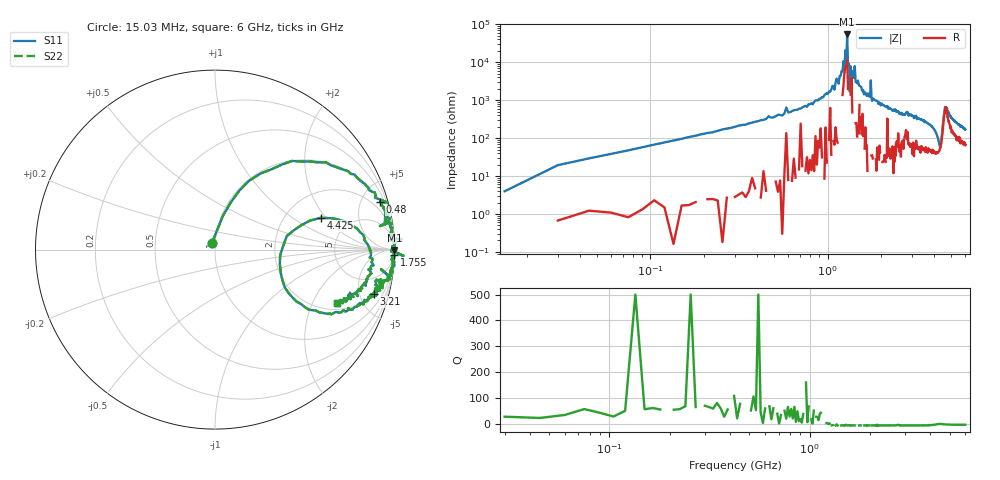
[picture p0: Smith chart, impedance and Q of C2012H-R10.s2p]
!	Network	Analyzer	HP8753E.07.74:	Oct	30	2002	Serial	No.	JP38451487
!	Hewlett-Packard
!	28	Aug	2009	10:31:47
!	Frequency	S11	S21	S12	S22
#	HZ	S	RI	R	50
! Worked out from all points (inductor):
!   400 points, 15.03 MHz to 6 GHz, reference 50 ohm
!   read as one part in series: L = 102 nH near 45.03 MHz
!   highest |Z| = 54.3 kohm at 1.29 GHz (marker M1)
!   self-resonance near 1.26 GHz
!   S11 on the Smith chart (normalised r, x): 15.03 MHz: 0.96, +0.07; 480 MHz: 1.10, +6.94; 1.755 GHz: 1, -67; 3.21 GHz: 2.08, -6.68; 4.425 GHz: 3.10, +1.76; 6 GHz: 2.34, -3.13
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1.502992e7  -0.017 0.0359  1.02 -0.0359  1.02 -0.0359  -0.017 0.0359
3.002985e7  0.042 0.184  0.958 -0.184  0.958 -0.184  0.042 0.184
1.050295e8  0.318 0.449  0.682 -0.449  0.682 -0.449  0.318 0.449
4.800276e8  0.92 0.264  0.0797 -0.264  0.0797 -0.264  0.92 0.264
1.020025e9  0.993 0.0584  0.00656 -0.0584  0.00656 -0.0584  0.993 0.0584
1.245024e9  0.982 6.1e-05  0.0183 -6.1e-05  0.0183 -6.1e-05  0.982 6.1e-05
1.260024e9  0.998 0.00443  0.00186 -0.00443  0.00186 -0.00443  0.998 0.00443
1.275024e9  1.01 -0.00208  -0.0123 0.00208  -0.0123 0.00208  1.01 -0.00208
1.290024e9  1 -0.0018  0.000397 0.0018  0.000397 0.0018  1 -0.0018
1.335023e9  1.05 -0.0352  -0.0513 0.0352  -0.0513 0.0352  1.05 -0.0352
1.350023e9  0.998 -0.0125  0.00244 0.0125  0.00244 0.0125  0.998 -0.0125
1.605022e9  1 -0.0703  -0.00238 0.0703  -0.00238 0.0703  1 -0.0703
1.755021e9  0.999 -0.0299  0.000855 0.0299  0.000855 0.0299  0.999 -0.0299
1.785021e9  0.986 -0.102  0.0144 0.102  0.0144 0.102  0.986 -0.102
2.01002e9  0.982 -0.122  0.0179 0.122  0.0179 0.122  0.982 -0.122
3.015015e9  0.92 -0.228  0.0804 0.228  0.0804 0.228  0.92 -0.228
3.210014e9  0.886 -0.247  0.114 0.247  0.114 0.247  0.886 -0.247
4.00501e9  0.695 -0.351  0.305 0.351  0.305 0.351  0.695 -0.351
4.425008e9  0.588 0.177  0.412 -0.177  0.412 -0.177  0.588 0.177
4.605007e9  0.865 -0.00366  0.135 0.00366  0.135 0.00366  0.865 -0.00366
5.010005e9  0.838 -0.188  0.162 0.188  0.162 0.188  0.838 -0.188
6e9  0.681 -0.299  0.319 0.299  0.319 0.299  0.681 -0.299
